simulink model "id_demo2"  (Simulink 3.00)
settings: Solver=ode45  SolverMode=SingleTasking  StartTime=0.0  StopTime=10  RelTol=1e-3  AbsTol=1e-3
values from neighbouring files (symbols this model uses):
  Au = [a0 a1;a2]    [data_id1.m]    (also in data_id2.m = [a0;[a1 a2]])
  Ay = [A0 A1;A2]    [data_id1.m]    (also in data_id2.m = A0)
  Bu = [b0;b1]    [data_id1.m]    (also in data_id2.m)
  By = [B0;B1]    [data_id1.m]    (also in data_id2.m)
  Cu = [c0 c1]/den(1)    [data_id1.m]    (also in data_id2.m = [c0 c1])
  Cy = [C0;C1]/den(1)    [data_id1.m]    (also in data_id2.m = [C0;C1])
  Du = zeros(in*(cit+1),in)    [data_id1.m]    (also in data_id2.m = zeros(cit*in,in))
  Dy = -[zeros(out,out);By]/den(1)    [data_id1.m]    (also in data_id2.m = [D1;D2])
libraries: simulink3 x1

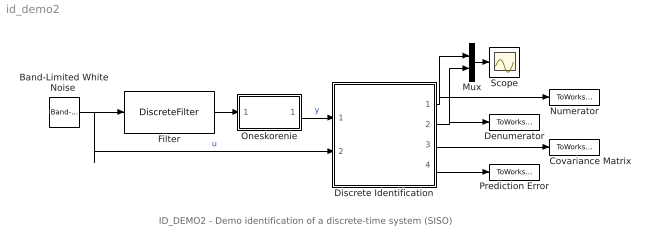
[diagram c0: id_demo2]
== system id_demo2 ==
  note: ID_DEMO2 - Demo identification of a discrete-time system (SISO)
  "Band-Limited White Noise " : simulink3/Sources/Band-Limited White Noise  Cov=[0.1]  Ts=0.1  seed=[23341]
  Covariance Matrix : ToWorkspace  VariableName=CovMatrix  SampleTime=0  SaveFormat=Matrix
  Denumerator : ToWorkspace  VariableName=A  SampleTime=0  SaveFormat=Matrix
  Discrete Identification : Subsystem  mask(Discrete Identification){par1=[2,2], Ds=[0], par2=[0.985,0.01], poc=[0 0 0 0], kov=[10e6], ts=[1]}
      mask prompts: par1 "Degrees of numerator and denominator -  [dn, dd]:"; Ds "Discrete time delay - [D]:"; par2 "Exponential forgetting and Bittanti's correction - [L, d]:"; poc "Initial parameter estimates - [theta(1) ... theta(n)]:"; kov "Covariance matrix (see help, standard - [10e6]):"; ts "Sampling time - [ts]:"
      mask help: Discrete identification Authors: Lubos Cirka and Miroslav Fikar 1998 - 2004
      mask init:
      | cit=par1(1);men=par1(2);L=par2(1);d=par2(2);n=cit+men;m=1;in=1;out=1;eval('data_id2');
  Filter : DiscreteFilter  Numerator=[0 0.8 0.2]  Denominator=[1 -0.5 0.06]  SampleTime=1
  Mux : Mux  Inputs=2
  Numerator : ToWorkspace  VariableName=B  SampleTime=0  SaveFormat=Matrix
  Oneskorenie : Subsystem  mask(Time Delay){LDd=[0], LDts=[1]}
      mask prompts: LDd "Discrete time delay - [D]:"; LDts "Sampling time - [ts]:"
      mask help: Discrete time delay Authors: Lubos Cirka and Miroslav Fikar 1998 - 2004
      mask init:
      | A=[zeros(1,1+LDd);eye(LDd),zeros(LDd,1)];B=[1;zeros(LDd,1)]; if LDd==0; C=0; D=1; else C=[zeros(1,LDd-1) 1 0]; D=0; end;
  Prediction Error : ToWorkspace  VariableName=PredError  SampleTime=0  SaveFormat=Matrix
  Scope : Scope
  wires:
  Oneskorenie/1(u(k-d)) -> Discrete Identification/1(y)  "y"
  "Band-Limited White Noise "/1 -> Filter/1, Discrete Identification/2(u)  "u"
  Mux/1 -> Scope/1
  Filter/1 -> Oneskorenie/1(u(k))
  Discrete Identification/4(prediction error) -> Prediction Error/1
  Discrete Identification/3("Covariance matrix ") -> Covariance Matrix/1
  Discrete Identification/2(A) -> Denumerator/1, Mux/2
  Discrete Identification/1(B) -> Mux/1, Numerator/1

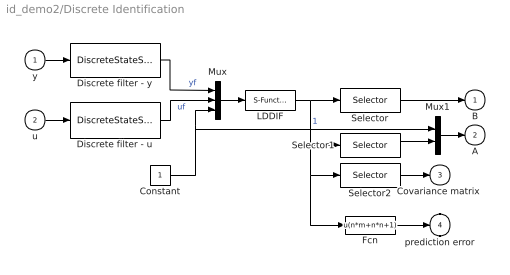
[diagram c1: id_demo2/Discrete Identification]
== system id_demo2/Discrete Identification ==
  y : Inport  Port=1  PortWidth=-1  SampleTime=-1  DataType=auto
  u : Inport  Port=2  PortWidth=-1  SampleTime=-1  DataType=auto
  Constant : Constant  Value=1
  Discrete filter - u : DiscreteStateSpace  A=Au  B=Bu  C=Cu  D=Du  X0=0  SampleTime=ts
  Discrete filter - y : DiscreteStateSpace  A=Ay  B=By  C=Cy  D=Dy  X0=0  SampleTime=ts
  Fcn : Fcn  Expr=u(n*m+n*n+1)
  LDDIF : S-Function  FunctionName=lddif_s  Parameters=m ,n+1 ,L ,d, [poc 0], kov, ts  PortCounts=[]  SFunctionModules=''
  Mux : Mux  Inputs=3
  Mux1 : Mux  Inputs=2
  Selector : Selector  Elements=[men+1:1:men+cit]  InputPortWidth=(n+1)*m+(n+1)*(n+1)+m
  Selector1 : Selector  Elements=[1:1:men]  InputPortWidth=(n+1)*m+(n+1)*(n+1)+m
  Selector2 : Selector  Elements=[(n+1)*m+1:1:(n+1)*m+(n+1)*(n+1)]  InputPortWidth=(n+1)*m+(n+1)*(n+1)+m
  B : Outport  Port=1  InitialOutput=0
  A : Outport  Port=2  InitialOutput=0
  "Covariance matrix " : Outport  Port=3  InitialOutput=0
  prediction error : Outport  Port=4  InitialOutput=0
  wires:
  LDDIF/1 -> Fcn/1, Selector2/1, Selector1/1, Selector/1
  Discrete filter - u/1 -> Mux/2  "uf"
  Discrete filter - y/1 -> Mux/1  "yf"
  u/1 -> Discrete filter - u/1
  y/1 -> Discrete filter - y/1
  Selector/1 -> B/1
  Mux/1 -> LDDIF/1
  Mux1/1 -> A/1
  Selector2/1 -> "Covariance matrix "/1
  Fcn/1 -> prediction error/1
  Selector1/1 -> Mux1/2
  Constant/1 -> Mux/3, Mux1/1  "1"

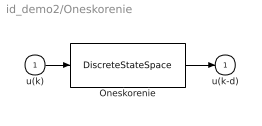
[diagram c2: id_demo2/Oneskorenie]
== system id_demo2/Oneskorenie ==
  u(k) : Inport  Port=1  PortWidth=-1  SampleTime=-1  DataType=auto
  Oneskorenie : DiscreteStateSpace  A=A  B=B  C=C  D=D  X0=0  SampleTime=LDts
  u(k-d) : Outport  Port=1  InitialOutput=0
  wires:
  Oneskorenie/1 -> u(k-d)/1
  u(k)/1 -> Oneskorenie/1
